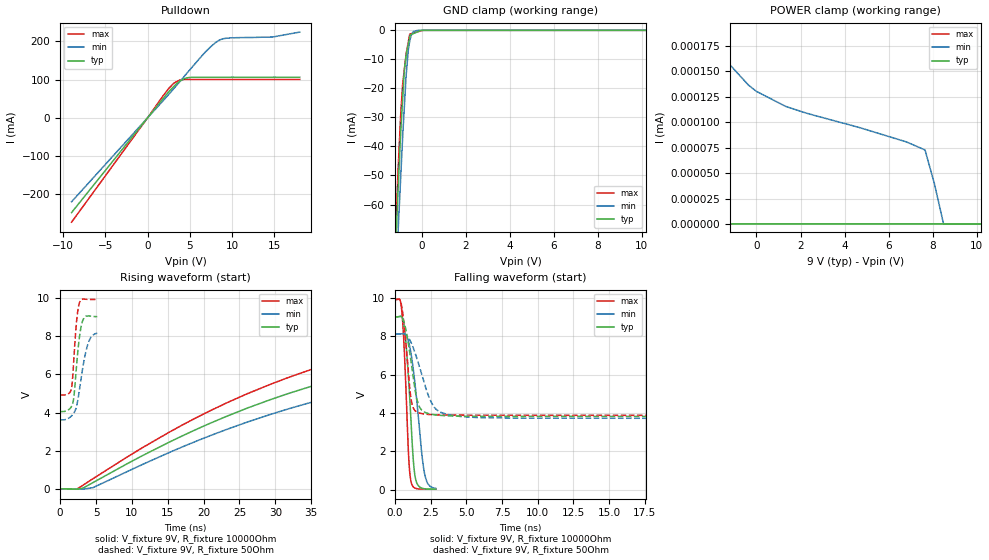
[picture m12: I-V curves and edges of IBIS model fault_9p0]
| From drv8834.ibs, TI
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|   fault_9p0 Model
[Model]   fault_9p0
Model_type   Open_drain
Polarity   Inverting
Vmeas = 4.5
Vref = 9
Cref = 2pF
Rref = 10000
|   typ   min   max
|   (nom PVT)   (fast PVT)   (slow PVT)
|C_comp from frequency sweep method (F = 125KHz)
|C_comp   2.234e-09   4.402e-10   2.501e-09
|ON state : BUFFER OUTPUT TURNED LOW
|C_comp   2.234e-09   4.402e-10   2.501e-09
|OFF state: BUFFER IN HIGH IMPEDANCE
|C_comp   3.292e-12   3.074e-12   3.519e-12
|C_comp from LC tank measurement(L=1nH)
|Resonant Frequency(Hz)   4.260e+09   4.280e+09   4.100e+09
 C_comp   1.397e-12   1.384e-12   1.508e-12
|ON state : BUFFER OUTPUT TURNED LOW
|Resonant Frequency(Hz)   4.260e+09   4.280e+09   4.100e+09
|C_comp   1.397e-12   1.384e-12   1.508e-12
|OFF state: BUFFER IN HIGH IMPEDANCE
|Resonant Frequency(Hz)   3.390e+09   3.460e+09   3.330e+09
|C_comp   2.206e-12   2.118e-12   2.287e-12
| Where nom  PVT is Nominal Process, 9V, 27C
|   Fast PVT is Strong Process,  9.9V, -40C
|   Slow PVT is Weak Process,   8.1V, 125C
[Voltage Range]   9   8.1   9.9
|Ambient Temperature   25   150   -40
|Junction Temperature
[Temperature Range]   27   125   -40
[Pullup Reference]   9   8.1   9.9
[Pulldown Reference]   0   0   0
[Power Clamp Reference]   9   8.1   9.9
[GND Clamp Reference]   0   0   0
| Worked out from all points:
|   slope of the pulldown table from 0 to 1.35 V, typ, clamps not added: 36.4 ohm
|   GND clamp passes 1 mA (typ) near -0.33 V on its own axis
|   falling waveform, V_fixture 9V, R_fixture 10000Ohm: 20-80 % time 441ps typ, 668ps min, 334ps max; typ from 9 V to 0.04 V
|   rising waveform, V_fixture 9V, R_fixture 10000Ohm: 20-80 % time 44.8ns typ, 47.3ns min, 41.3ns max; typ from 0.033 V to 8.97 V
|   falling waveform, V_fixture 9V, R_fixture 50Ohm: 20-80 % time 602ps typ, 1.21ns min, 372ps max; typ from 9 V to 4.05 V
|   rising waveform, V_fixture 9V, R_fixture 50Ohm: 20-80 % time 744ps typ, 1.22ns min, 572ps max; typ from 4.05 V to 9 V
[Pulldown]
|   Voltage   I(typ)   I(min)   I(max)
-9V       -247.9mA   -219.6mA   -273mA
1.742V    47.82mA    42.44mA    54.82mA
2.505V    68.2mA     61.27mA    77.02mA
3.158V    83.13mA    77.84mA    91.26mA
3.812V    95.65mA    94.69mA    98.7mA
4.698V    104.5mA    117.9mA    100.3mA
6.812V    106.1mA    171.4mA    100.3mA
7.654V    106.1mA    189.5mA    100.3mA
8.497V    106.1mA    203.1mA    100.3mA
9.769V    106.1mA    208.8mA    100.3mA
14.81V    106.1mA    211.3mA    100.3mA
18V       106.1mA    224.1mA    100.3mA
[GND Clamp]
|   Voltage   I(typ)   I(min)   I(max)
-9V       -1.59A     -1.902A    -1.667A
-1.197V   -78.47mA   -91.48mA   -73.62mA
-1.079V   -57.49mA   -71.7mA    -50.74mA
-1.053V   -52.85mA   -67.38mA   -46.19mA
-950.4mV  -35.87mA   -51.3mA    -29.54mA
-861.3mV  -24.14mA   -37.39mA   -18.98mA
-774mV    -13.25mA   -25.46mA   -13.09mA
-696.6mV  -8.414mA   -15.28mA   -8.058mA
-599.4mV  -4.747mA   -6.728mA   -3.97mA
-513mV    -1.57mA    -2.988mA   -1.253mA
-364.5mV  -1.107mA   -379.7uA   -922.1uA
18V       0A         0A         0A
[POWER Clamp]
|   Voltage   I(typ)   I(min)   I(max)
-9V       4.147mA    4.174mA    5.727mA
-2.583V   46.23uA    200.8uA    204.4nA
-2.475V   7.214uA    139.3uA    0A
-2.357V   187.7nA    77.55uA    0A
-2.295V   13.69nA    48.82uA    0A
-2.276V   0A         40.58uA    0A
-2.041V   0A         461.7nA    0A
-1.207V   0A         156.4nA    0A
-50.39fV  0A         130.2nA    0A
7.654V    0A         72.67nA    0A
8.497V    0A         0A         0A
18V       0A         0A         0A
[Ramp]
R_load = 10000
|   typ   min   max
dV/dt_r   5.38045/4.50826e-08   4.83938/4.78122e-08   5.92104/4.13417e-08
dV/dt_f   5.38045/4.41249e-10   4.83938/6.72584e-10   5.92104/3.34633e-10
[Falling Waveform]
V_fixture = 9V
V_fixture_min = 8.1V
V_fixture_max = 9.9V
R_fixture = 10000Ohm
C_fixture = 0F
|   Time   V(typ)   V(min)   V(max)
0s        9V         8.099V     9.9V
325ps     9.023V     8.102V     9.907V
500ps     8.944V     8.118V     9.041V
775ps     7.507V     8.022V     4.976V
950ps     5.688V     7.681V     1.719V
1.1ns     3.783V     7.153V     486.7mV
1.3ns     1.334V     6.117V     141.3mV
1.5ns     398.7mV    4.784V     66.5mV
2.075ns   55.27mV    817.2mV    39.78mV
2.85ns    40.07mV    76.47mV    36.93mV
[Rising Waveform]
V_fixture = 9V
V_fixture_min = 8.1V
V_fixture_max = 9.9V
R_fixture = 10000Ohm
C_fixture = 0F
|   Time   V(typ)   V(min)   V(max)
0s        32.57mV    33.06mV    31.59mV
2.4ns     10.99mV    12.53mV    37.05mV
4.575ns   352mV      89.58mV    555.1mV
19.27ns   3.175V     2.557V     3.793V
31.42ns   4.947V     4.151V     5.776V
46.32ns   6.463V     5.546V     7.444V
58.23ns   7.283V     6.319V     8.339V
73.68ns   7.981V     7.005V     9.075V
92.47ns   8.47V      7.507V     9.548V
165.2ns   8.974V     8.059V     9.889V
[Falling Waveform]
V_fixture = 9V
V_fixture_min = 8.1V
V_fixture_max = 9.9V
R_fixture = 50Ohm
C_fixture = 0F
|   Time   V(typ)   V(min)   V(max)
0s        9V         8.1V       9.9V
325ps     9.013V     8.102V     9.898V
475ps     8.978V     8.109V     9.5V
725ps     8.431V     8.078V     7.869V
1.05ns    7.016V     7.769V     5.122V
1.325ns   5.59V      7.279V     4.188V
1.75ns    4.256V     6.306V     3.987V
2.7ns     3.915V     4.342V     3.909V
4.525ns   3.835V     3.822V     3.887V
1.101us   4.051V     3.618V     4.911V
[Rising Waveform]
V_fixture = 9V
V_fixture_min = 8.1V
V_fixture_max = 9.9V
R_fixture = 50Ohm
C_fixture = 0F
|   Time   V(typ)   V(min)   V(max)
0s        4.051V     3.618V     4.918V
1.175ns   4.15V      3.711V     4.99V
1.6ns     4.335V     3.832V     5.295V
1.9ns     4.789V     3.971V     6.722V
2.275ns   6.384V     4.308V     8.698V
2.725ns   8.034V     5.283V     9.764V
3.15ns    8.804V     6.333V     9.919V
3.825ns   9.034V     7.518V     9.905V
4.4ns     9.023V     7.989V     9.9V
5.175ns   9.003V     8.138V     9.899V
